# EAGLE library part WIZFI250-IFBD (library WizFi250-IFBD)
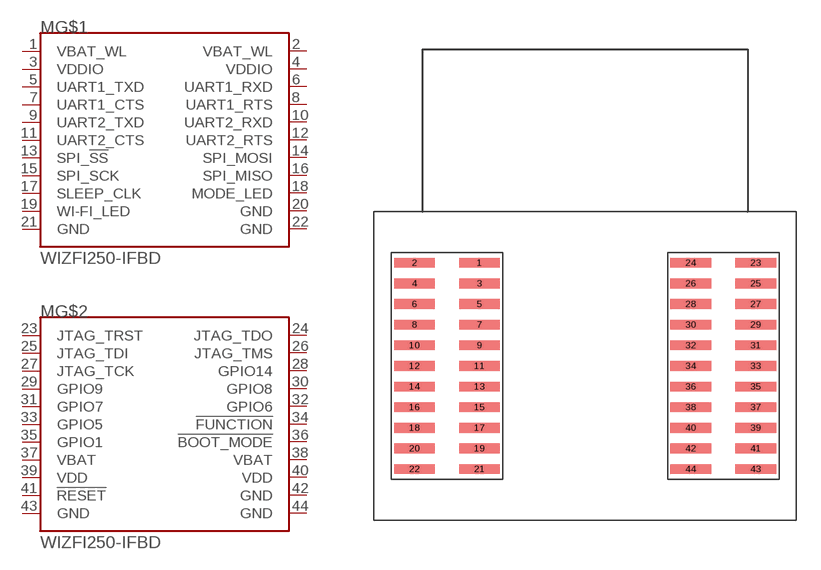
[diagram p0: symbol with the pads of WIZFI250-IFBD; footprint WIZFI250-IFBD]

Designator prefix M; gates G$1=WIZFI250-IFBD-1 G$2=WIZFI250-IFBD-2

## WIZFI250-IFBD  [WIZFI250-IFBD]
1  G$1:VBAT_WL  pas
2  G$1:VBAT_WL  pas
3  G$1:VDDIO  pas
4  G$1:VDDIO  pas
5  G$1:UART1_TXD  pas
6  G$1:UART1_RXD  pas
7  G$1:UART1_CTS  pas
8  G$1:UART1_RTS  pas
9  G$1:UART2_TXD  pas
10  G$1:UART2_RXD  pas
11  G$1:UART2_CTS  pas
12  G$1:UART2_RTS  pas
13  G$1:SPI_!SS  pas
14  G$1:SPI_MOSI  pas
15  G$1:SPI_SCK  pas
16  G$1:SPI_MISO  pas
17  G$1:SLEEP_CLK  pas
18  G$1:MODE_LED  pas
19  G$1:WI-FI_LED  pas
20  G$1:GND  pas
21  G$1:GND  pas
22  G$1:GND  pas
23  G$2:JTAG_TRST  pas
24  G$2:JTAG_TDO  pas
25  G$2:JTAG_TDI  pas
26  G$2:JTAG_TMS  pas
27  G$2:JTAG_TCK  pas
28  G$2:GPIO14  pas
29  G$2:GPIO9  pas
30  G$2:GPIO8  pas
31  G$2:GPIO7  pas
32  G$2:GPIO6  pas
33  G$2:GPIO5  pas
34  G$2:!FUNCTION  pas
35  G$2:GPIO1  pas
36  G$2:!BOOT_MODE  pas
37  G$2:VBAT  pas
38  G$2:VBAT  pas
39  G$2:VDD  pas
40  G$2:VDD  pas
41  G$2:!RESET  pas
42  G$2:GND  pas
43  G$2:GND  pas
44  G$2:GND  pas

## Footprint WIZFI250-IFBD (pad centres in mm)
smd 2.5 x 0.6: 1 -6.5,6.35; 2 -10.5,6.35; 3 -6.5,5.08; 4 -10.5,5.08; 5 -6.5,3.81; 6 -10.5,3.81; 7 -6.5,2.54; 8 -10.5,2.54; 9 -6.5,1.27; 10 -10.5,1.27; 11 -6.5,0; 12 -10.5,0; 13 -6.5,-1.27; 14 -10.5,-1.27; 15 -6.5,-2.54; 16 -10.5,-2.54; 17 -6.5,-3.81; 18 -10.5,-3.81; 19 -6.5,-5.08; 20 -10.5,-5.08; 21 -6.5,-6.35; 22 -10.5,-6.35; 23 10.5,6.35; 24 6.5,6.35; 25 10.5,5.08; 26 6.5,5.08; 27 10.5,3.81; 28 6.5,3.81; 29 10.5,2.54; 30 6.5,2.54; 31 10.5,1.27; 32 6.5,1.27; 33 10.5,0; 34 6.5,0; 35 10.5,-1.27; 36 6.5,-1.27; 37 10.5,-2.54; 38 6.5,-2.54; 39 10.5,-3.81; 40 6.5,-3.81; 41 10.5,-5.08; 42 6.5,-5.08; 43 10.5,-6.35; 44 6.5,-6.35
